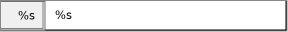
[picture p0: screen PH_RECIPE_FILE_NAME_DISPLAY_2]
VISUALIZATION PH_RECIPE_FILE_NAME_DISPLAY_2  // 288x32
VAR_IN_OUT
	RECIPE_CTRL_V2 : ST_RecipeCtrl_2;
END_VAR
VAR_INPUT
	IDX : UDINT;
END_VAR
VAR_INPUT
	Right_Edge_Rel : INT;
END_VAR
    Rectangle (0,0 286x30), input disabled if: TRUE, colour variable: RECIPE_CTRL_V2.sStatus.asFileDisplay[IDX].b32FillColor
        p874137650: Right_Edge_Rel
    Rectangle (45,1 238x28), "%s", text variable: RECIPE_CTRL_V2.sStatus.asFileDisplay[IDX].sgFilesName, input disabled if: RECIPE_CTRL_V2.sStatus.asFileDisplay[IDX].sgFilesName = '' OR RECIPE_CTRL_V2.sStatus.bBusy
        p874137650: Right_Edge_Rel
        p55702900: RECIPE_CTRL_V2.sStatus.asFileDisplay[IDX].b32TextColor
        OnMouseUp: execute { RECIPE_CTRL_V2.u32RecipeNum:=(RECIPE_CTRL_V2.sStatus.asFileDisplay[IDX].u32Index); }
    Button (0,1 45x29), "%s", text variable: RECIPE_CTRL_V2.sStatus.asFileDisplay[IDX].u32Index, input disabled if: TRUE
        p55702900: RECIPE_CTRL_V2.sStatus.asFileDisplay[IDX].b32TextColor
END_VISUALIZATION
